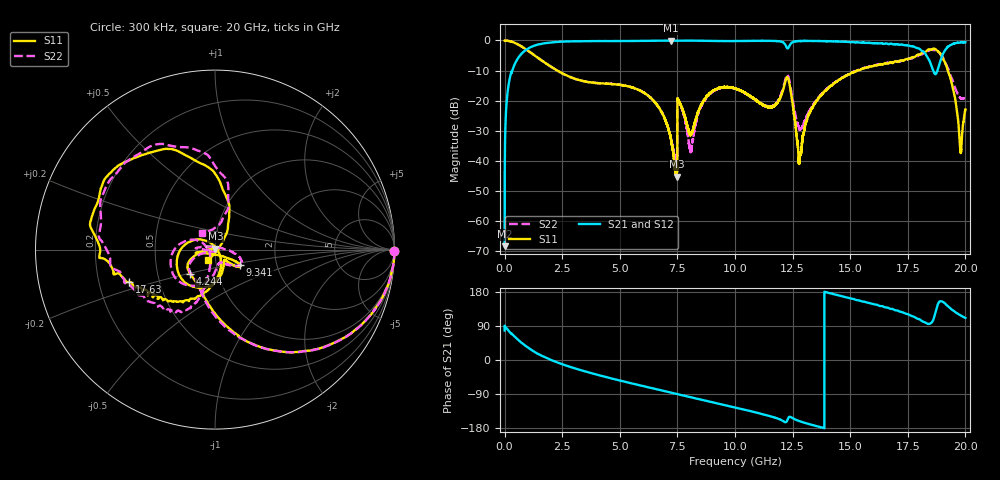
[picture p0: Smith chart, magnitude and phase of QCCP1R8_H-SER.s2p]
!{QCCP1R8}
!Johanson Technology Inc.
!www.johansontechnology.com
!Test Board Conditions:
!Substrate Type  RO4350B
!Substrate Thickness  20 mil
!Substrate Dk  3.66
!TL Type: GCPW
!TL Trace Width  36 mil
!TL Gap  12 mil
!Electrode orientation  Horizontal
!DUT TOPOLOGY	SERIES
!Mounting Pad LxW  26x36 mil
! Created Sat Jan  9 18:26:04 2021
# hz S ma R 50
! 2 Port Network Data from SP1.SP block
! freq  magS11  angS11  magS21  angS21  magS12  angS12  magS22  angS22
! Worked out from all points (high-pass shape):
!   20001 points, 300 kHz to 20 GHz, reference 50 ohm
!   highest |S21| = -0.04 dB at 7.228 GHz (marker M1); lowest = -68.2 dB at 300 kHz (marker M2)
!   |S21| within 3 dB of the highest: 944.2 MHz to 18.05 GHz (17.1 GHz wide, 180 % of centre); 19.14 GHz to end of sweep
!   lowest |S11| = -45.2 dB at 7.467 GHz (marker M3), VSWR 1.01, Z = 50.2 + j0.524 ohm
!   |S11| at or under -10 dB: 2.29 GHz to 15.28 GHz (12.99 GHz wide, 148 % of centre); 19.24 GHz to end of sweep
!   |S22| runs from -40.1 to 0.0 dB; largest |S21 - S12| = 0.016
!   S11 on the Smith chart (normalised r, x): 300 kHz: open; 4.244 GHz: 0.73, -0.21; 9.341 GHz: 1.30, -0.23; 17.63 GHz: 0.33, -0.16; 20 GHz: 0.91, -0.11
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300000  0.9946 -0.3  0.0003875 77.9  0.0003163 80.6  0.9964 -0.4
1.333e8  0.9894 -9.6  0.1423 80.1  0.1422 80.2  0.9888 -9.6
4.993e8  0.8904 -31.4  0.4485 58.2  0.4484 58.2  0.8917 -31.5
1.6583e9  0.453 -79.0  0.8881 9.8  0.8866 9.9  0.4519 -80.7
3.3343e9  0.2154 -117.7  0.9731 -27.3  0.9727 -27.3  0.2152 -116.5
4.2443e9  0.194 -135.0  0.9758 -42.5  0.9763 -42.5  0.1936 -129.4
6.6673e9  0.08032 -169.3  0.9909 -78.1  0.991 -78.2  0.07923 -162.9
7.2283e9  0.02224 173.0  0.9954 -86.1  0.9938 -86.1  0.02259 -150.5
7.4673e9  0.00552 71.2  0.9932 -89.5  0.9931 -89.5  0.01177 -71.8
7.6003e9  0.093 -168.5  0.9899 -91.6  0.9887 -91.5  0.09163 171.4
8.0823e9  0.02732 -96.9  0.9924 -98.3  0.9924 -98.3  0.01458 82.7
9.3413e9  0.1629 -31.3  0.9781 -115.8  0.9792 -115.9  0.1611 -23.3
1.00003e10  0.1585 -36.9  0.9786 -125.1  0.9794 -125.2  0.1589 -34.6
1.15283e10  0.07898 -48.9  0.9825 -148.2  0.9838 -148.3  0.07954 -70.4
1.22823e10  0.2452 -143.7  0.7369 -157.2  0.7353 -157.2  0.2686 -154.1
1.28063e10  0.01021 20.3  0.9765 -161.5  0.9781 -161.5  0.03366 -165.4
1.33343e10  0.07513 -62.7  0.9799 -171.0  0.9794 -171.1  0.07863 -109.0
1.66673e10  0.4195 -142.8  0.8695 137.2  0.8751 136.6  0.4215 -126.0
1.76253e10  0.5095 -159.3  0.8014 117.3  0.8068 117.0  0.4998 -152.8
1.88783e10  0.629 117.0  0.4119 154.5  0.4118 153.7  0.6124 110.6
1.97753e10  0.01575 -11.1  0.925 118.2  0.9248 118.2  0.1117 99.3
2e10  0.0716 -126.8  0.9367 110.9  0.9357 110.9  0.1174 129.0
